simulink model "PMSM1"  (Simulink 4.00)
settings: Solver=ode45  StartTime=-eps  StopTime=0.2  FixedStep=0.000001  RelTol=1e-3
undefined symbols (not defined in the file or in its folder): di, Element, J, Lsx, Lsy, p, Psim, Rs, sfunxy, Symmetrized, Ts, Udc, Warning
libraries: simulink3 x1

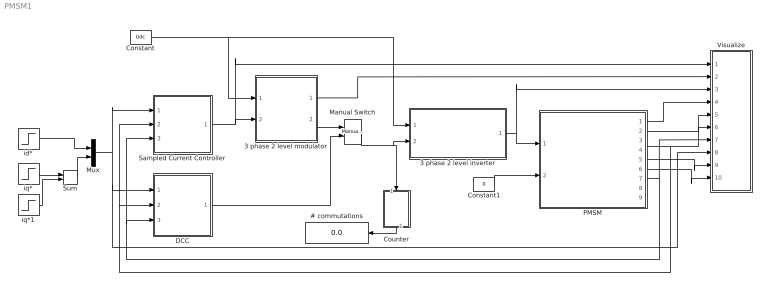
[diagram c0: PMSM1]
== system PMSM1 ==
  # commutations : Display
  3 phase 2 level inverter : Subsystem
  3 phase 2 level modulator : Subsystem  mask{type=Symmetrized, Random=Fixed frequency, Ts=Ts}
      mask prompts: type "Sinus, Symmetrized or Minimum switch modulation"; Random "Fixed or random modulation?"; Ts "Sampling interval"
      mask help: Carrier Wave modulator that uses either fixed frequency modulation or random modulation. The fixed frequency modulation uses 1/(2Ts) as modulation frequency. The random modulation selects the modulatio frequency by random every sampling instant. The selection uses either 1/Ts, 1/(2Ts) or 1/(3Ts) as carrier wave frequency.
  Constant : Constant  Value=Udc
  Constant1 : Constant  Value=0
  Counter : Subsystem  Orientation=down
  DCC : Subsystem
  Manual Switch : simulink3/Nonlinear/Manual Switch  sw=1  action=0
  Mux : Mux  Inputs=2
  PMSM : Subsystem  mask{Psim=Psim, p=p, Rs=Rs, isy=[0 1], psisy=[0 Lsy], isx=[0 1], psisx=[0 Lsx], J=J}
      mask prompts: p "Number of poles"; Rs "Stator resistance"; isy "y-axis current vector"; psisy "y-axis flux vector"; isx "x-axis current vector"; psisx "x-axis flux vector"; J "Inertia"
  Sampled Current Controller : Subsystem  mask{R=Rs, Lx=Lsx, Ly=Lsy, Kp=[(Lsx/Ts+Rs/2) (Lsy/Ts+Rs/2)]', Ti=[(Lsx/Rs+Ts/2) (Lsy/Rs+Ts/2)]', Ts=Ts, Umax=Udc, Umin=-Udc, SlowFast=Fast computer}
      mask prompts: R "Load resistance"; Lx "x-axis load inductance"; Ly "y-axis load inductance"; Kp "Controller gain"; Ti "Integral Time Constant"; Ts "Sampling time [s]"; Umax "Max output signal"; Umin "Min output signal"; SlowFast "Controller type"
  Sum : Sum  Inputs=++  SaturateOnIntegerOverflow=on
  Visualize : Subsystem
  id* : Step  Time=0.0105  Before=0  After=0  SampleTime=0
  iq* : Step  Time=0.0055  Before=0  After=10  SampleTime=0
  iq*1 : Step  Time=0.05  Before=0  After=-5  SampleTime=0
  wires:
  3 phase 2 level inverter/1(va,b,c) -> Visualize/3(v), PMSM/1(vabc)
  Sampled Current Controller/1(u*) -> 3 phase 2 level modulator/2(uabc*), Visualize/1(u*)
  Constant/1 -> 3 phase 2 level inverter/1(Udc), 3 phase 2 level modulator/1(Udc)
  Counter/1(#) -> # commutations/1
  3 phase 2 level modulator/2(sa,b,c) -> Manual Switch/1
  Manual Switch/1 -> 3 phase 2 level inverter/2(sa,b,c), Counter/1(sa,b,c)
  DCC/1(sa,b,c) -> Manual Switch/2
  3 phase 2 level modulator/1(mod) -> Visualize/2(mod)
  id*/1 -> Mux/1
  Mux/1 -> Sampled Current Controller/1(Ref_dq), DCC/1(Ref_dq), Visualize/8(i*dq)
  PMSM/7(theta_el) -> Visualize/7(theta), Sampled Current Controller/3(thetaR), DCC/3(thetaR)
  Constant1/1 -> PMSM/2(Tl)
  PMSM/1(uabc) -> Visualize/4("u ")
  PMSM/4(is) -> Visualize/6(i), DCC/2(Act_ab), Sampled Current Controller/2(Act_ab)
  PMSM/2(exy) -> Visualize/5(e)
  PMSM/5(T_mech) -> Visualize/9(Tmech)
  PMSM/6(w_mech) -> Visualize/10(wmech)
  iq*/1 -> Sum/1
  iq*1/1 -> Sum/2
  Sum/1 -> Mux/2

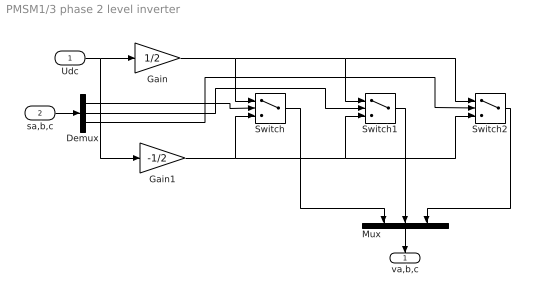
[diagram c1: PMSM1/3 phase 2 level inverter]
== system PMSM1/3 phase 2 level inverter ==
  Udc : Inport  Port=1  LatchInput=off
  sa,b,c : Inport  Port=2  LatchInput=off
  Demux : Demux  Outputs=3  BusSelectionMode=off
  Gain : Gain  Gain=1/2  Multiplication=Element-wise(K.*u)  SaturateOnIntegerOverflow=on
  Gain1 : Gain  Gain=-1/2  Multiplication=Element-wise(K.*u)  SaturateOnIntegerOverflow=on
  Mux : Mux  Orientation=down  Inputs=3
  Switch : Switch  Threshold=0
  Switch1 : Switch  Threshold=0
  Switch2 : Switch  Threshold=0
  va,b,c : Outport  Orientation=down  Port=1  InitialOutput=0
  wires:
  Gain/1 -> Switch/1, Switch1/1, Switch2/1
  Gain1/1 -> Switch/3, Switch1/3, Switch2/3
  Udc/1 -> Gain1/1, Gain/1
  sa,b,c/1 -> Demux/1
  Demux/1 -> Switch/2
  Demux/2 -> Switch1/2
  Demux/3 -> Switch2/2
  Switch/1 -> Mux/1
  Switch1/1 -> Mux/2
  Switch2/1 -> Mux/3
  Mux/1 -> va,b,c/1

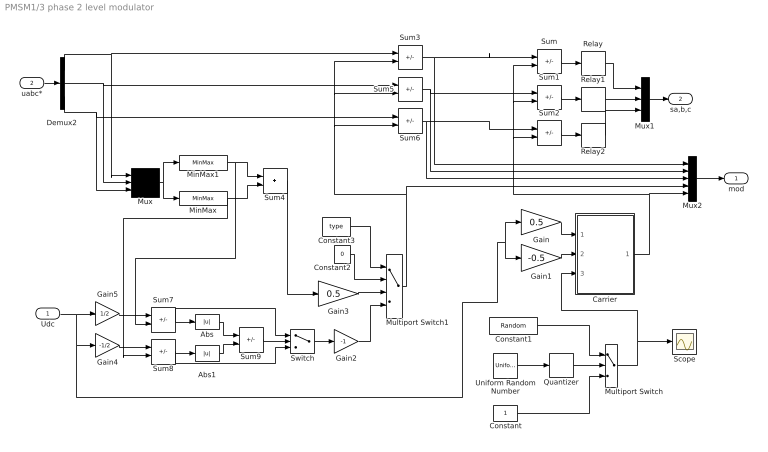
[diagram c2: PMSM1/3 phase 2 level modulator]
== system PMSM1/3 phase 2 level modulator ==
  Udc : Inport  Port=1  LatchInput=off
  uabc* : Inport  Port=2  LatchInput=off
  Abs : Abs  SaturateOnIntegerOverflow=on
  Abs1 : Abs  SaturateOnIntegerOverflow=on
  Carrier : Subsystem
  Constant : Constant  Value=1
  Constant1 : Constant  Value=Random
  Constant2 : Constant  Value=0
  Constant3 : Constant  Value=type
  Demux2 : Demux  Outputs=3  BusSelectionMode=off
  Gain : Gain  Gain=0.5  Multiplication=Element-wise(K.*u)  SaturateOnIntegerOverflow=on
  Gain1 : Gain  Gain=-0.5  Multiplication=Element-wise(K.*u)  SaturateOnIntegerOverflow=on
  Gain2 : Gain  Gain=-1  Multiplication=Element-wise(K.*u)  SaturateOnIntegerOverflow=on
  Gain3 : Gain  Gain=0.5  Multiplication=Element-wise(K.*u)  SaturateOnIntegerOverflow=on
  Gain4 : Gain  Gain=-1/2  Multiplication=Element-wise(K.*u)  SaturateOnIntegerOverflow=on
  Gain5 : Gain  Gain=1/2  Multiplication=Element-wise(K.*u)  SaturateOnIntegerOverflow=on
  MinMax : MinMax  Function=min  Inputs=1
  MinMax1 : MinMax  Function=max  Inputs=1
  Multiport Switch : MultiPortSwitch  Inputs=2
  Multiport Switch1 : MultiPortSwitch  Inputs=3
  Mux : Mux  Inputs=3
  Mux1 : Mux  Inputs=3
  Mux2 : Mux  Inputs=5
  Quantizer : Quantizer  QuantizationInterval=1  LinearizeAsGain=on
  Relay : Relay  OnSwitchValue=eps  OffSwitchValue=eps  OnOutputValue=1  OffOutputValue=-1
  Relay1 : Relay  OnSwitchValue=eps  OffSwitchValue=eps  OnOutputValue=1  OffOutputValue=-1
  Relay2 : Relay  OnSwitchValue=eps  OffSwitchValue=eps  OnOutputValue=1  OffOutputValue=-1
  Scope : Scope
  Sum{,1..3,5..8} (8 alike) : Sum  Inputs=+-  SaturateOnIntegerOverflow=on
  Sum4 : Sum  Inputs=++  SaturateOnIntegerOverflow=on
  Sum9 : Sum  Inputs=-+  SaturateOnIntegerOverflow=on
  Switch : Switch  Threshold=0
  Uniform Random Number : UniformRandomNumber  Minimum=1  Maximum=3  Seed=0.9874  SampleTime=Ts
  mod : Outport  Port=1  InitialOutput=0
  sa,b,c : Outport  Port=2  InitialOutput=0
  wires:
  Carrier/1(um) -> Sum2/2, Sum1/2, Sum/2, Mux2/5
  Gain1/1 -> Carrier/2(Umin)
  Gain/1 -> Carrier/1(Umax)
  Sum/1 -> Relay/1
  Relay1/1 -> Mux1/2
  Sum1/1 -> Relay1/1
  Relay2/1 -> Mux1/3
  Sum2/1 -> Relay2/1
  Quantizer/1 -> Multiport Switch/2
  Uniform Random Number/1 -> Quantizer/1
  Constant/1 -> Multiport Switch/3
  Multiport Switch/1 -> Carrier/3(x), Scope/1
  Constant1/1 -> Multiport Switch/1
  Sum3/1 -> Mux2/1, Sum/1
  Sum5/1 -> Mux2/2, Sum1/1
  Sum6/1 -> Mux2/3, Sum2/1
  Demux2/1 -> Sum3/1, Mux/1
  Demux2/2 -> Sum5/1, Mux/2
  Demux2/3 -> Sum6/1, Mux/3
  Mux/1 -> MinMax1/1, MinMax/1
  MinMax1/1 -> Sum4/1, Sum7/2
  MinMax/1 -> Sum4/2, Sum8/2
  Udc/1 -> Gain5/1, Gain4/1, Gain1/1, Gain/1
  Gain4/1 -> Sum8/1
  Sum7/1 -> Abs/1, Switch/1
  Sum8/1 -> Abs1/1, Switch/3
  Abs/1 -> Sum9/1
  Abs1/1 -> Sum9/2
  Sum9/1 -> Switch/2
  Sum4/1 -> Gain3/1
  Switch/1 -> Gain2/1
  Constant3/1 -> Multiport Switch1/1
  Constant2/1 -> Multiport Switch1/2
  Gain3/1 -> Multiport Switch1/3
  Gain2/1 -> Multiport Switch1/4
  Multiport Switch1/1 -> Sum5/2, Sum3/2, Sum6/2, Mux2/4
  Gain5/1 -> Sum7/1
  uabc*/1 -> Demux2/1
  Relay/1 -> Mux1/1
  Mux1/1 -> sa,b,c/1
  Mux2/1 -> mod/1

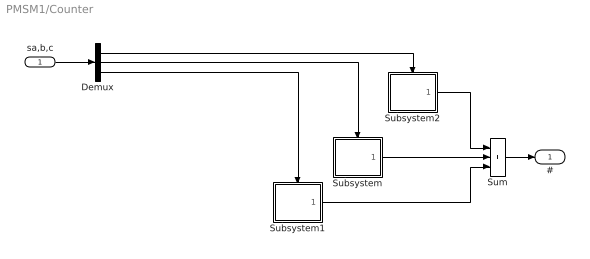
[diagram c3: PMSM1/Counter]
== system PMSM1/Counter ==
  sa,b,c : Inport  Port=1  LatchInput=off
  Demux : Demux  Outputs=3  BusSelectionMode=off
  Subsystem : Subsystem  TreatAsAtomicUnit=on
  Subsystem1 : Subsystem  TreatAsAtomicUnit=on
  Subsystem2 : Subsystem  TreatAsAtomicUnit=on
  Sum : Sum  Inputs=+++  SaturateOnIntegerOverflow=on
  # : Outport  Port=1
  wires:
  Sum/1 -> #/1
  Subsystem/1(Out1) -> Sum/2
  Subsystem2/1(Out1) -> Sum/1
  Subsystem1/1(Out1) -> Sum/3
  sa,b,c/1 -> Demux/1
  Demux/2 -> Subsystem/Trigger
  Demux/3 -> Subsystem1/Trigger
  Demux/1 -> Subsystem2/Trigger

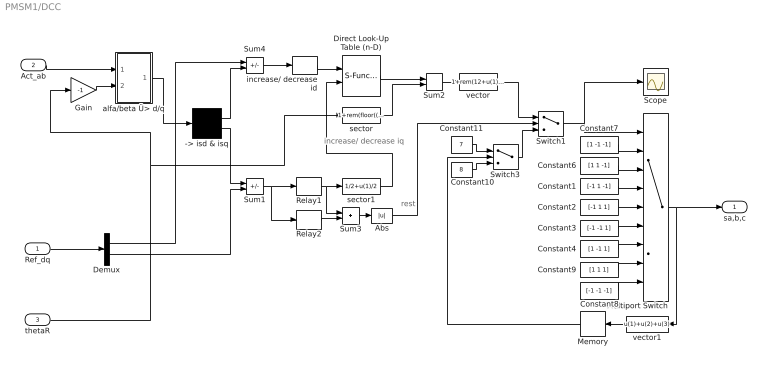
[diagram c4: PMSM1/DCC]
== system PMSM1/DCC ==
  note: increase/ decrease iq
  note: rest
  Ref_dq : Inport  Port=1  LatchInput=off
  Act_ab : Inport  Port=2  LatchInput=off
  thetaR : Inport  Port=3  LatchInput=off
  -> isd & isq : Demux  Outputs=2  BusSelectionMode=off
  Abs : Abs  SaturateOnIntegerOverflow=on
  Constant1 : Constant  Value=[-1 1 -1]
  Constant10 : Constant  Value=8
  Constant11 : Constant  Value=7
  Constant2 : Constant  Value=[-1 1 1]
  Constant3 : Constant  Value=[-1 -1 1]
  Constant4 : Constant  Value=[1 -1 1]
  Constant6 : Constant  Value=[1 1 -1]
  Constant7 : Constant  Value=[1 -1 -1]
  Constant8 : Constant  Value=[-1 -1 -1]
  Constant9 : Constant  Value=[1 1 1]
  Demux : Demux  Outputs=2  BusSelectionMode=off
  Direct Look-Up Table (n-D) : S-Function  FunctionName=sfun_nddirectlook  Parameters=numInputs,mxTable,clipFlag,tabIsInput,numTDims  PortCounts=[]  SFunctionModules=''  mask(LookupNDDirect){maskTabDims=2, explicitNumDims=1, outDims=Element, tabIsInput=off, mxTable=[4 2;5 1], clipFlag=Warning}
      mask prompts: maskTabDims "Number of table dimensions:"; explicitNumDims "Explicit number of table dimensions:"; outDims "Inputs select this object from table:"; tabIsInput "Make table an input"; mxTable "Table data:"; clipFlag "Action for out of range input:"
      mask help: Table member selection. Inputs are zero-based indices into the table, e.g., an input of 3 returns the fourth element in that dimension. Block can also be used to select a column or 2-D matrix out of the table.
      mask init:
      | if tabIsInput == 1
      |   tWhat = ' T';
      |   yT = 1/(3+maskTabDims-outDims);
      | else
      |   tWhat = ' ';
      |   yT = 0;
      | end
      | if maskTabDims >= 5
      |   numTDims = explicitNumDims;
      | else
      |   numTDims = maskTabDims;
      | end
      | numInputs =  numTDims - (outDims-1);
      | if strcmp(get_param(bdroot(gcb),'BlockDiagramType'),'library')
      |   dimsChar = 'n';
      | else
      |   dimsChar = sprintf('%d',numTDims);
      | end
      | [x,y] = nddirectico('plotdata', numTDims, tabIsInput, outDims);
      | xp = x((end-3):end); yp = y((end-3):end);
      | x = x(1:(end-4)); y = y(1:(end-4));
  Gain : Gain  Gain=-1  Multiplication=Element-wise(K.*u)  SaturateOnIntegerOverflow=on
  Memory : Memory  Orientation=left  X0=0  InheritSampleTime=off
  Multiport Switch : MultiPortSwitch  Inputs=8
  Relay1 : Relay  OnSwitchValue=di/2  OffSwitchValue=-di/2  OnOutputValue=1  OffOutputValue=-1
  Relay2 : Relay  OnSwitchValue=1.3*di/2  OffSwitchValue=-1.3*di/2  OnOutputValue=1  OffOutputValue=-1
  Scope : Scope
  Sum1 : Sum  Inputs=-+  SaturateOnIntegerOverflow=on
  Sum2 : Sum  Inputs=++  SaturateOnIntegerOverflow=on
  Sum3 : Sum  Inputs=++  SaturateOnIntegerOverflow=on
  Sum4 : Sum  Inputs=+-  SaturateOnIntegerOverflow=on
  Switch1 : Switch  Threshold=1
  Switch3 : Switch  Threshold=1
  alfa/beta Ü> d/q : Subsystem
  increase/ decrease id : Relay  OnSwitchValue=di/2  OffSwitchValue=-di/2  OnOutputValue=1  OffOutputValue=0
  sector : Fcn  Expr=1+rem(floor((2*pi+u(1)+pi/6)/(pi/3+eps)),6)
  sector1 : Fcn  Expr=1/2+u(1)/2
  vector : Fcn  Expr=1+rem(12+u(1)-1,6)
  vector1 : Fcn  Orientation=left  Expr=u(1)+u(2)+u(3)
  sa,b,c : Outport  Port=1
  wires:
  Gain/1 -> alfa/beta Ü> d/q/2(angle)
  Act_ab/1 -> alfa/beta Ü> d/q/1(vect)
  alfa/beta Ü> d/q/1(Out) -> -> isd & isq/1
  -> isd & isq/1 -> Sum4/2
  Multiport Switch/1 -> vector1/1, sa,b,c/1
  Switch1/1 -> Multiport Switch/1, Scope/1
  vector/1 -> Switch1/1
  Sum4/1 -> increase/ decrease id/1
  Sum2/1 -> vector/1
  vector1/1 -> Memory/1
  -> isd & isq/2 -> Sum1/1
  Constant10/1 -> Switch3/3
  Constant11/1 -> Switch3/1
  Memory/1 -> Switch3/2
  Switch3/1 -> Switch1/3
  Relay1/1 -> Sum3/1, sector1/1
  Relay2/1 -> Sum3/2
  Sum3/1 -> Abs/1
  Sum1/1 -> Relay1/1, Relay2/1
  Abs/1 -> Switch1/2
  increase/ decrease id/1 -> Direct Look-Up Table (n-D)/1
  sector1/1 -> Direct Look-Up Table (n-D)/2
  sector/1 -> Sum2/2
  Direct Look-Up Table (n-D)/1 -> Sum2/1
  Constant6/1 -> Multiport Switch/3
  Constant7/1 -> Multiport Switch/2
  Constant8/1 -> Multiport Switch/9
  Constant9/1 -> Multiport Switch/8
  Constant1/1 -> Multiport Switch/4
  Constant2/1 -> Multiport Switch/5
  Constant3/1 -> Multiport Switch/6
  Constant4/1 -> Multiport Switch/7
  Ref_dq/1 -> Demux/1
  Demux/1 -> Sum4/1
  Demux/2 -> Sum1/2
  thetaR/1 -> Gain/1, sector/1

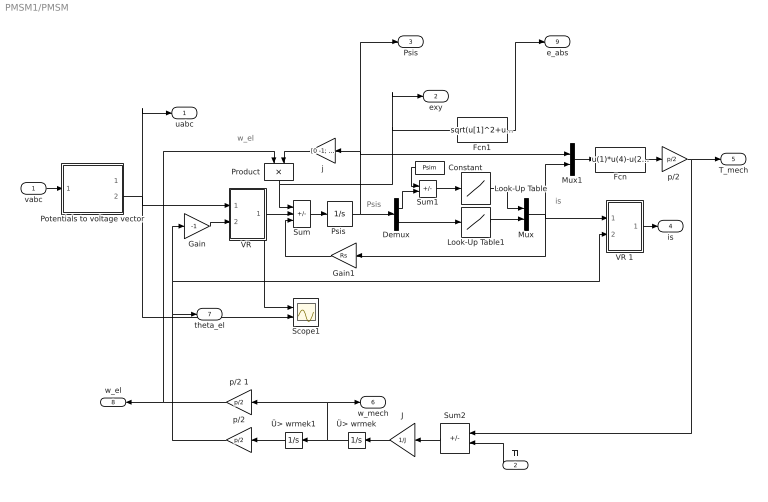
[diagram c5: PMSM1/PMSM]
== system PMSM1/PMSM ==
  note: w_el
  note: Psis
  note: is
  vabc : Inport  Port=1  LatchInput=off
  Tl : Inport  Orientation=left  Port=2  LatchInput=off
  Constant : Constant  Orientation=left  Value=Psim
  Demux : Demux  Outputs=2  BusSelectionMode=off
  Fcn : Fcn  Expr=u(1)*u(4)-u(2)*u(3)
  Fcn1 : Fcn  Expr=sqrt(u[1]^2+u[2]^2)
  Gain : Gain  Gain=-1  Multiplication=Element-wise(K.*u)  SaturateOnIntegerOverflow=on
  Gain1 : Gain  Orientation=left  Gain=Rs  Multiplication=Element-wise(K.*u)  SaturateOnIntegerOverflow=on
  J : Gain  Orientation=left  Gain=1/J  Multiplication=Element-wise(K.*u)  SaturateOnIntegerOverflow=on
  Look-Up Table : Lookup  InputValues=psisx  OutputValues=isx
  Look-Up Table1 : Lookup  InputValues=psisy  OutputValues=isy
  Mux : Mux  Inputs=2
  Mux1 : Mux  Inputs=2
  Potentials to voltage vector : Subsystem
  Product : Product  Orientation=down  Inputs=2  Multiplication=Element-wise(.*)  SaturateOnIntegerOverflow=on
  "Psis " : Integrator  ExternalReset=none  InitialConditionSource=internal  InitialCondition=[Psim 0]'  LimitOutput=on  UpperSaturationLimit=[2*Psim Psim*2]'  LowerSaturationLimit=[Psim/20 0]'  ShowSaturationPort=off  ShowStatePort=off  AbsoluteTolerance=auto
  Scope1 : Scope  NumInputPorts=2
  Sum : Sum  Inputs=-+-  SaturateOnIntegerOverflow=on
  Sum1 : Sum  Inputs=-+  SaturateOnIntegerOverflow=on
  Sum2 : Sum  Orientation=left  Inputs=+-  SaturateOnIntegerOverflow=on
  "VR " : Subsystem
  VR 1 : Subsystem
  j : Gain  Orientation=left  Gain=[0 -1; 1 0]  Multiplication=Matrix(K*u)  SaturateOnIntegerOverflow=on
  p/2 : Gain  Orientation=left  Gain=p/2  Multiplication=Matrix(K*u)  SaturateOnIntegerOverflow=on
  "p/2 " : Gain  Gain=p/2  Multiplication=Matrix(K*u)  SaturateOnIntegerOverflow=on
  p/2 1 : Gain  Orientation=left  Gain=p/2  Multiplication=Matrix(K*u)  SaturateOnIntegerOverflow=on
  Ü> wrmek : Integrator  Orientation=left  ExternalReset=none  InitialConditionSource=internal  InitialCondition=0  LimitOutput=off  UpperSaturationLimit=inf  LowerSaturationLimit=-inf  ShowSaturationPort=off  ShowStatePort=off  AbsoluteTolerance=auto
  Ü> wrmek1 : Integrator  Orientation=left  ExternalReset=none  InitialConditionSource=internal  InitialCondition=0  LimitOutput=off  UpperSaturationLimit=inf  LowerSaturationLimit=-inf  ShowSaturationPort=off  ShowStatePort=off  AbsoluteTolerance=auto
  uabc : Outport  Port=1
  exy : Outport  Port=2
  Psis : Outport  Port=3
  is : Outport  Port=4
  T_mech : Outport  Port=5
  w_mech : Outport  Port=6
  theta_el : Outport  Port=7
  w_el : Outport  Orientation=left  Port=8
  e_abs : Outport  Port=9
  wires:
  VR 1/1(Out) -> is/1
  Ü> wrmek/1 -> Ü> wrmek1/1, p/2 1/1, w_mech/1
  Fcn1/1 -> e_abs/1
  p/2 1/1 -> w_el/1, Product/1
  Tl/1 -> Sum2/2
  Ü> wrmek1/1 -> p/2/1
  Sum2/1 -> J/1
  J/1 -> Ü> wrmek/1
  vabc/1 -> Potentials to voltage vector/1(In1)
  Potentials to voltage vector/2(uab) -> "VR "/1(vect), uabc/1, Scope1/2
  "p/2 "/1 -> Sum2/1, T_mech/1
  Gain/1 -> "VR "/2(angle)
  Sum/1 -> "Psis "/1
  "Psis "/1 -> Demux/1, j/1, Mux1/1, Psis/1
  Demux/1 -> Sum1/2
  Demux/2 -> Look-Up Table1/1
  Look-Up Table/1 -> Mux/1
  Look-Up Table1/1 -> Mux/2
  Mux/1 -> Mux1/2, Gain1/1, VR 1/1(vect)
  Mux1/1 -> Fcn/1
  Constant/1 -> Sum1/1
  Sum1/1 -> Look-Up Table/1
  Gain1/1 -> Sum/3
  "VR "/1(Out) -> Sum/2, Scope1/1
  Product/1 -> Sum/1, Fcn1/1, exy/1
  Fcn/1 -> "p/2 "/1
  j/1 -> Product/2
  p/2/1 -> theta_el/1, Gain/1, VR 1/2(angle)

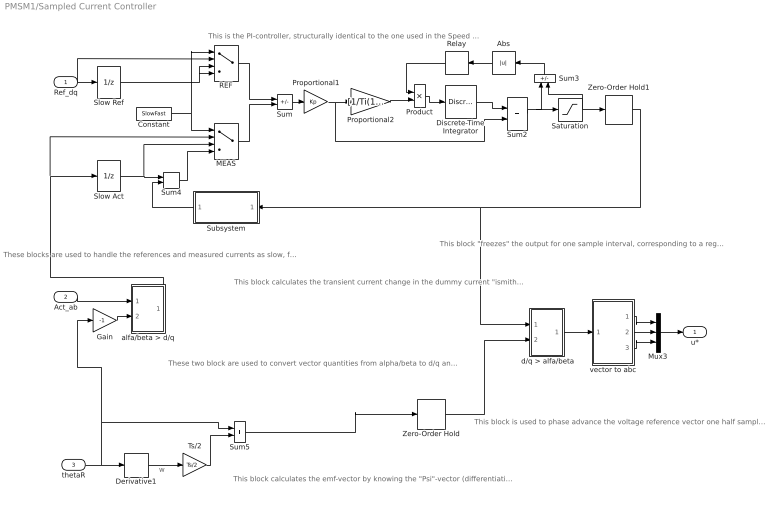
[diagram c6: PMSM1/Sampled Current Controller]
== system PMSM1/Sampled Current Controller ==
  note: These blocks are used to handle the references and measured currents as slow, fast or fast computer with Smith predictor.
  note: This block calculates the transient current change in the dummy current "ismith" The smith predictor calculates the current change that would have been measured if the computer was "fast", i.e. without the delay that a slow computer has. The calculated current change equals the real current change, but informing the controller one sampling interval earlier, thus allowing a high (deadbeat) gain.
  note: This is the PI-controller, structurally identical to the one used in the Speed Controller
  note: This block "freezes" the output for one sample interval, corresponding to a register in a microcontroller where the reference voltages are written once every sampling inteval.
  note: These two block are used to convert vector quantities from alpha/beta to d/q and back again. Note that they are identical, but use the angle with opposite sign.
  note: This block calculates the emf-vector by knowing the "Psi"-vector (differentiation) and calculates the emf- components in the d/q-plane (ideally there is only "eq" whilse "ed"=0). It alse calculates the angle of the "Psi"- vector, used to orient the d/q-plane.
  note: This block is used to phase advance the voltage reference vector one half sample period. It is done to compensate for the fact that the "reality" is turning during the same sample period as the voltage references are being held constant. In the beginning of the sample period, the voltage reference will be 1/2 sample period ahead of reality, and in the end of the sample period it will be 1/2 period behind. In average, it will be in the correct position relative to reality.
  note: w
  Ref_dq : Inport  Port=1  LatchInput=off
  Act_ab : Inport  Port=2  LatchInput=off
  thetaR : Inport  Port=3  LatchInput=off
  " d/q > alfa/beta" : Subsystem
  Abs : Abs  Orientation=left  SaturateOnIntegerOverflow=on
  Constant : Constant  Value=SlowFast
  Derivative1 : Derivative
  Discrete-Time Integrator : DiscreteIntegrator  IntegratorMethod=ForwardEuler  ExternalReset=none  InitialConditionSource=internal  InitialCondition=0  LimitOutput=on  UpperSaturationLimit=Umax  LowerSaturationLimit=Umin  ShowSaturationPort=off  ShowStatePort=off  SampleTime=Ts
  Gain : Gain  Gain=-1  Multiplication=Element-wise(K.*u)  SaturateOnIntegerOverflow=on
  MEAS : MultiPortSwitch  Inputs=3
  Mux3 : Mux  Inputs=3
  Product : Product  Inputs=2  Multiplication=Element-wise(.*)  SaturateOnIntegerOverflow=on
  Proportional1 : Gain  Gain=Kp  Multiplication=Element-wise(K.*u)  SaturateOnIntegerOverflow=on
  Proportional2 : Gain  Gain=[1/Ti(1) 1/Ti(2)]  Multiplication=Element-wise(K.*u)  SaturateOnIntegerOverflow=on
  REF : MultiPortSwitch  Inputs=3
  Relay : Relay  Orientation=left  OnSwitchValue=eps  OffSwitchValue=eps  OnOutputValue=0  OffOutputValue=1
  Saturation : Saturate  UpperLimit=Umax  LowerLimit=Umin  LinearizeAsGain=on
  Slow Act : UnitDelay  X0=0  SampleTime=Ts
  Slow Ref : UnitDelay  X0=0  SampleTime=Ts
  Subsystem : Subsystem  Orientation=left
  Sum : Sum  Inputs=+-  SaturateOnIntegerOverflow=on
  Sum2 : Sum  Inputs=++  SaturateOnIntegerOverflow=on
  Sum3 : Sum  Orientation=up  Inputs=+-  SaturateOnIntegerOverflow=on
  Sum4 : Sum  Inputs=++  SaturateOnIntegerOverflow=on
  Sum5 : Sum  Inputs=++  SaturateOnIntegerOverflow=on
  Ts/2 : Gain  Gain=Ts/2  Multiplication=Matrix(K*u)  SaturateOnIntegerOverflow=on
  Zero-Order Hold : ZeroOrderHold  SampleTime=Ts
  Zero-Order Hold1 : ZeroOrderHold  SampleTime=Ts
  alfa/beta > d/q : Subsystem
  vector to abc : Subsystem
  u* : Outport  Port=1
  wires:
  Discrete-Time Integrator/1 -> Sum2/1
  Proportional1/1 -> Proportional2/1, Sum2/2
  Sum/1 -> Proportional1/1
  Sum2/1 -> Saturation/1, Sum3/1
  Saturation/1 -> Zero-Order Hold1/1, Sum3/2
  Proportional2/1 -> Product/2
  Product/1 -> Discrete-Time Integrator/1
  Relay/1 -> Product/1
  Ref_dq/1 -> REF/2, Slow Ref/1
  Zero-Order Hold1/1 -> Subsystem/1(u), " d/q > alfa/beta"/1(vect)
  Slow Act/1 -> Sum4/1, MEAS/3
  Subsystem/1(di_smith) -> Sum4/2
  Constant/1 -> MEAS/1, REF/1
  Slow Ref/1 -> REF/3, REF/4
  REF/1 -> Sum/1
  Sum4/1 -> MEAS/4
  MEAS/1 -> Sum/2
  Sum3/1 -> Abs/1
  Abs/1 -> Relay/1
  Gain/1 -> alfa/beta > d/q/2(angle)
  Act_ab/1 -> alfa/beta > d/q/1(vect)
  Sum5/1 -> Zero-Order Hold/1
  Zero-Order Hold/1 -> " d/q > alfa/beta"/2(angle)
  " d/q > alfa/beta"/1(Out) -> vector to abc/1(vect)
  vector to abc/1(a) -> Mux3/1
  vector to abc/2(b) -> Mux3/2
  vector to abc/3(c) -> Mux3/3
  alfa/beta > d/q/1(Out) -> Slow Act/1, MEAS/2
  Mux3/1 -> u*/1
  thetaR/1 -> Derivative1/1, Gain/1, Sum5/1
  Derivative1/1 -> Ts/2/1
  Ts/2/1 -> Sum5/2

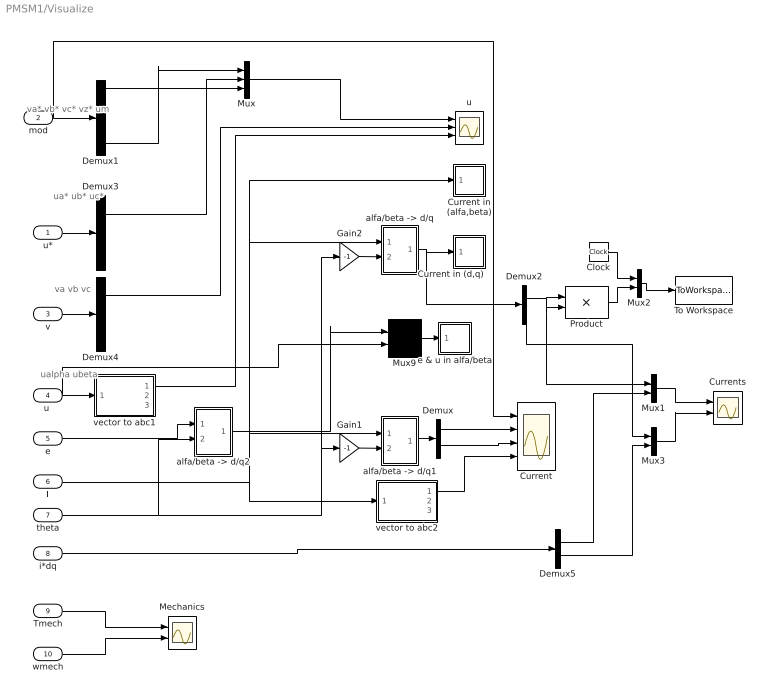
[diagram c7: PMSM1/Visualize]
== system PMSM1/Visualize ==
  note: va* vb* vc* vz* um
  note: ua* ub* uc*
  note: ualpha ubeta
  note: va vb vc
  u* : Inport  Port=1  LatchInput=off
  mod : Inport  Port=2  LatchInput=off
  v : Inport  Port=3  LatchInput=off
  "u " : Inport  Port=4  LatchInput=off
  e : Inport  Port=5  LatchInput=off
  i : Inport  Port=6  LatchInput=off
  theta : Inport  Port=7  LatchInput=off
  i*dq : Inport  Port=8  LatchInput=off
  Tmech : Inport  Port=9  LatchInput=off
  wmech : Inport  Port=10  LatchInput=off
  Clock : Clock
  Current : Scope  NumInputPorts=4
  Current in (alfa,beta) : Subsystem  LoadFcn=sfunxy([],[],[],'LoadBlock')  StartFcn=sfunxy([],[],[],'Start')  StopFcn=sfunxy([],[],[],'Stop')  mask(XY scope.){xmin=-20, xmax=20, ymin=-20, ymax=20, st=-1}
      mask prompts: xmin "x-min:"; xmax "x-max:"; ymin "y-min:"; ymax "y-max:"; st "Sample time:"
      mask help: XY scope using MATLAB graph window. First input is used as time base. Enter plotting ranges.
  Current in (d,q) : Subsystem  LoadFcn=sfunxy([],[],[],'LoadBlock')  StartFcn=sfunxy([],[],[],'Start')  StopFcn=sfunxy([],[],[],'Stop')  mask(XY scope.){xmin=-20, xmax=20, ymin=-20, ymax=20, st=-1}
      mask prompts: xmin "x-min:"; xmax "x-max:"; ymin "y-min:"; ymax "y-max:"; st "Sample time:"
      mask help: XY scope using MATLAB graph window. First input is used as time base. Enter plotting ranges.
  Currents : Scope  NumInputPorts=2
  Demux : Demux  Outputs=2  BusSelectionMode=off
  Demux1 : Demux  Outputs=5  BusSelectionMode=off
  Demux2 : Demux  Outputs=2  BusSelectionMode=off
  Demux3 : Demux  Outputs=3  BusSelectionMode=off
  Demux4 : Demux  Outputs=3  BusSelectionMode=off
  Demux5 : Demux  Outputs=2  BusSelectionMode=off
  Gain1 : Gain  Gain=-1  Multiplication=Element-wise(K.*u)  SaturateOnIntegerOverflow=on
  Gain2 : Gain  Gain=-1  Multiplication=Element-wise(K.*u)  SaturateOnIntegerOverflow=on
  Mechanics : Scope  NumInputPorts=2
  Mux : Mux  Inputs=3
  Mux{1..3,9} (4 alike) : Mux  Inputs=2
  Product : Product  Inputs=2  Multiplication=Element-wise(.*)  SaturateOnIntegerOverflow=on
  To Workspace : ToWorkspace  VariableName=f1  SampleTime=-1  SaveFormat=Array
  "alfa/beta -> d/q" : Subsystem
  "alfa/beta -> d/q1" : Subsystem
  "alfa/beta -> d/q2" : Subsystem
  e & u in alfa/beta : Subsystem  LoadFcn=sfunxy([],[],[],'LoadBlock')  StartFcn=sfunxy([],[],[],'Start')  StopFcn=sfunxy([],[],[],'Stop')  mask(XY scope.){xmin=-300, xmax=300, ymin=-300, ymax=300, st=-1}
      mask prompts: xmin "x-min:"; xmax "x-max:"; ymin "y-min:"; ymax "y-max:"; st "Sample time:"
      mask help: XY scope using MATLAB graph window. First input is used as time base. Enter plotting ranges.
  u : Scope  NumInputPorts=3
  vector to abc1 : Subsystem
  vector to abc2 : Subsystem
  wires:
  Gain2/1 -> "alfa/beta -> d/q"/2(angle)
  Gain1/1 -> "alfa/beta -> d/q1"/2(angle)
  "alfa/beta -> d/q1"/1(Out) -> Demux/1
  Demux/1 -> Current/2
  Demux/2 -> Current/3
  vector to abc2/1(a) -> Current/4
  mod/1 -> Demux1/1, Current/1
  "alfa/beta -> d/q"/1(Out) -> Current in (d,q)/1(xy), Demux2/1
  Demux1/5 -> Mux/1
  Demux1/1 -> Mux/3
  Mux/1 -> u/1
  u*/1 -> Demux3/1
  "u "/1 -> vector to abc1/1(vect), Mux9/2
  Demux3/1 -> Mux/2
  v/1 -> Demux4/1
  Demux4/1 -> u/2
  vector to abc1/1(a) -> u/3
  i/1 -> Current in (alfa,beta)/1(xy), "alfa/beta -> d/q"/1(vect), "alfa/beta -> d/q1"/1(vect), vector to abc2/1(vect)
  Mux9/1 -> e & u in alfa/beta/1(xy)
  theta/1 -> Gain1/1, Gain2/1, "alfa/beta -> d/q2"/2(angle)
  Clock/1 -> Mux2/1
  Product/1 -> Mux2/2
  Mux2/1 -> To Workspace/1
  Demux2/1 -> Product/1, Product/2, Mux1/1
  i*dq/1 -> Demux5/1
  Demux5/1 -> Mux1/2
  Demux2/2 -> Mux3/1
  Demux5/2 -> Mux3/2
  Mux3/1 -> Currents/2
  Mux1/1 -> Currents/1
  e/1 -> "alfa/beta -> d/q2"/1(vect)
  "alfa/beta -> d/q2"/1(Out) -> Mux9/1
  Tmech/1 -> Mechanics/1
  wmech/1 -> Mechanics/2

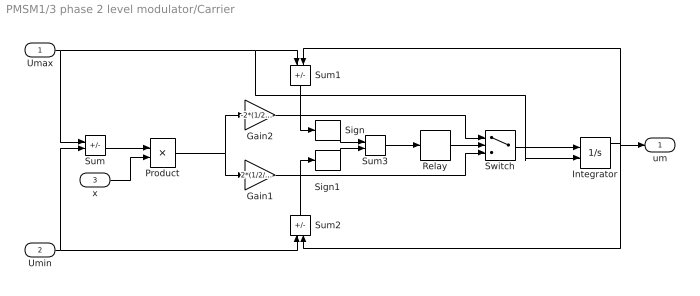
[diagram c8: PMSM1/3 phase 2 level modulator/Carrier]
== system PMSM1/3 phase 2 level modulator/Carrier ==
  Umax : Inport  Port=1  LatchInput=off
  Umin : Inport  Port=2  LatchInput=off
  x : Inport  Port=3  LatchInput=off
  Gain1 : Gain  Gain=2*(1/2/Ts)  Multiplication=Element-wise(K.*u)  SaturateOnIntegerOverflow=on
  Gain2 : Gain  Gain=-2*(1/2/Ts)  Multiplication=Element-wise(K.*u)  SaturateOnIntegerOverflow=on
  Integrator : Integrator  ExternalReset=none  InitialConditionSource=external  InitialCondition=0  LimitOutput=off  UpperSaturationLimit=inf  LowerSaturationLimit=-inf  ShowSaturationPort=off  ShowStatePort=off  AbsoluteTolerance=auto
  Product : Product  Inputs=2  Multiplication=Element-wise(.*)  SaturateOnIntegerOverflow=on
  Relay : Relay  OnSwitchValue=1  OffSwitchValue=-1  OnOutputValue=1  OffOutputValue=-1
  Sign : Signum
  Sign1 : Signum
  Sum : Sum  Inputs=+-  SaturateOnIntegerOverflow=on
  Sum1 : Sum  Orientation=down  Inputs=-+  SaturateOnIntegerOverflow=on
  Sum2 : Sum  Orientation=up  Inputs=-+  SaturateOnIntegerOverflow=on
  Sum3 : Sum  Inputs=++  SaturateOnIntegerOverflow=on
  Switch : Switch  Threshold=0
  um : Outport  Port=1
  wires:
  Switch/1 -> Integrator/1
  Umax/1 -> Sum/1, Sum1/1, Integrator/2
  Umin/1 -> Sum/2, Sum2/1
  Gain2/1 -> Switch/1
  Gain1/1 -> Switch/3
  Integrator/1 -> Sum1/2, um/1, Sum2/2
  Sum1/1 -> Sign/1
  Sum2/1 -> Sign1/1
  Sign/1 -> Sum3/1
  Sign1/1 -> Sum3/2
  Sum3/1 -> Relay/1
  Relay/1 -> Switch/2
  Sum/1 -> Product/1
  Product/1 -> Gain2/1, Gain1/1
  x/1 -> Product/2

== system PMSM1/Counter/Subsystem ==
  Trigger : TriggerPort  TriggerType=either  OutputDataType=auto
  Constant : Constant  Value=1
  Memory : Memory  Orientation=left  X0=0  InheritSampleTime=on
  Sum : Sum  Inputs=++  SaturateOnIntegerOverflow=on
  Out1 : Outport  Port=1
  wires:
  Sum/1 -> Memory/1, Out1/1
  Memory/1 -> Sum/2
  Constant/1 -> Sum/1

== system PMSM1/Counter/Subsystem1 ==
  Trigger : TriggerPort  TriggerType=either  OutputDataType=auto
  Constant : Constant  Value=1
  Memory : Memory  Orientation=left  X0=0  InheritSampleTime=on
  Sum : Sum  Inputs=++  SaturateOnIntegerOverflow=on
  Out1 : Outport  Port=1
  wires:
  Constant/1 -> Sum/1
  Memory/1 -> Sum/2
  Sum/1 -> Memory/1, Out1/1

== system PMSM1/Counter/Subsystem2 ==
  Trigger : TriggerPort  TriggerType=either  OutputDataType=auto
  Constant : Constant  Value=1
  Memory : Memory  Orientation=left  X0=0  InheritSampleTime=on
  Sum : Sum  Inputs=++  SaturateOnIntegerOverflow=on
  Out1 : Outport  Port=1
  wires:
  Sum/1 -> Memory/1, Out1/1
  Memory/1 -> Sum/2
  Constant/1 -> Sum/1

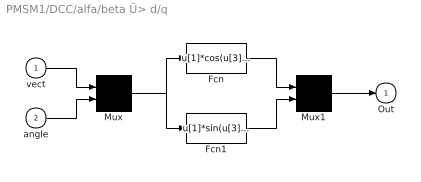
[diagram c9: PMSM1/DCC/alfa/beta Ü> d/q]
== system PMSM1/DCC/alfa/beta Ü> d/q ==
  vect : Inport  Port=1  LatchInput=off
  angle : Inport  Port=2  LatchInput=off
  Fcn : Fcn  Expr=u[1]*cos(u[3])-u[2]*sin(u[3])
  Fcn1 : Fcn  Expr=u[1]*sin(u[3])+u[2]*cos(u[3])
  Mux : Mux  Inputs=2
  Mux1 : Mux  Inputs=2
  Out : Outport  Port=1  InitialOutput=0
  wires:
  vect/1 -> Mux/1
  angle/1 -> Mux/2
  Mux/1 -> Fcn/1, Fcn1/1
  Fcn/1 -> Mux1/1
  Fcn1/1 -> Mux1/2
  Mux1/1 -> Out/1

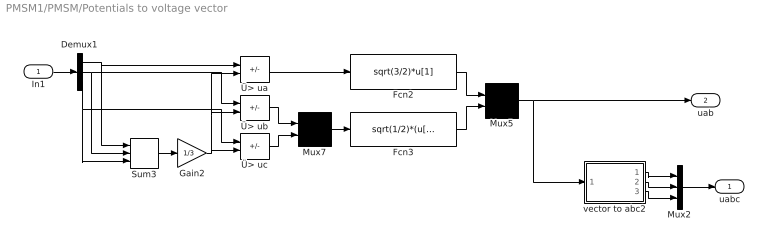
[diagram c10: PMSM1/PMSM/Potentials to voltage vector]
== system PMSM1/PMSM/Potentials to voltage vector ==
  In1 : Inport  Port=1  LatchInput=off
  Demux1 : Demux  Outputs=3  BusSelectionMode=off
  Fcn2 : Fcn  Expr=sqrt(3/2)*u[1]
  Fcn3 : Fcn  Expr=sqrt(1/2)*(u[1]-u[2])
  Gain2 : Gain  Gain=1/3  Multiplication=Element-wise(K.*u)  SaturateOnIntegerOverflow=on
  Mux2 : Mux  Inputs=3
  Mux5 : Mux  Inputs=2
  Mux7 : Mux  Inputs=2
  Sum3 : Sum  Inputs=+++  SaturateOnIntegerOverflow=on
  vector to abc2 : Subsystem
  Ü> ua : Sum  Inputs=+-  SaturateOnIntegerOverflow=on
  Ü> ub : Sum  Inputs=+-  SaturateOnIntegerOverflow=on
  Ü> uc : Sum  Inputs=+-  SaturateOnIntegerOverflow=on
  uabc : Outport  Port=1
  uab : Outport  Port=2
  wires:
  Fcn3/1 -> Mux5/2
  Fcn2/1 -> Mux5/1
  Mux7/1 -> Fcn3/1
  Ü> uc/1 -> Mux7/2
  Ü> ub/1 -> Mux7/1
  Ü> ua/1 -> Fcn2/1
  Gain2/1 -> Ü> uc/2, Ü> ub/2, Ü> ua/2
  Demux1/2 -> Ü> ub/1, Sum3/2
  Sum3/1 -> Gain2/1
  Demux1/3 -> Ü> uc/1, Sum3/3
  Demux1/1 -> Ü> ua/1, Sum3/1
  In1/1 -> Demux1/1
  Mux5/1 -> uab/1, vector to abc2/1(vect)
  vector to abc2/1(a) -> Mux2/1
  vector to abc2/2(b) -> Mux2/2
  vector to abc2/3(c) -> Mux2/3
  Mux2/1 -> uabc/1

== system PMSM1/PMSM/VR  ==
  vect : Inport  Port=1  LatchInput=off
  angle : Inport  Port=2  LatchInput=off
  Fcn : Fcn  Expr=u[1]*cos(u[3])-u[2]*sin(u[3])
  Fcn1 : Fcn  Expr=u[1]*sin(u[3])+u[2]*cos(u[3])
  Mux : Mux  Inputs=2
  Mux1 : Mux  Inputs=2
  Out : Outport  Port=1  InitialOutput=0
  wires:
  Mux1/1 -> Out/1
  Fcn1/1 -> Mux1/2
  Fcn/1 -> Mux1/1
  Mux/1 -> Fcn1/1, Fcn/1
  angle/1 -> Mux/2
  vect/1 -> Mux/1

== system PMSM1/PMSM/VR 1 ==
  vect : Inport  Port=1  LatchInput=off
  angle : Inport  Port=2  LatchInput=off
  Fcn : Fcn  Expr=u[1]*cos(u[3])-u[2]*sin(u[3])
  Fcn1 : Fcn  Expr=u[1]*sin(u[3])+u[2]*cos(u[3])
  Mux : Mux  Inputs=2
  Mux1 : Mux  Inputs=2
  Out : Outport  Port=1  InitialOutput=0
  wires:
  vect/1 -> Mux/1
  angle/1 -> Mux/2
  Mux/1 -> Fcn/1, Fcn1/1
  Fcn/1 -> Mux1/1
  Fcn1/1 -> Mux1/2
  Mux1/1 -> Out/1

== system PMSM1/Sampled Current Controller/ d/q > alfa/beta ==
  vect : Inport  Port=1  LatchInput=off
  angle : Inport  Port=2  LatchInput=off
  Fcn : Fcn  Expr=u[1]*cos(u[3])-u[2]*sin(u[3])
  Fcn1 : Fcn  Expr=u[1]*sin(u[3])+u[2]*cos(u[3])
  Mux : Mux  Inputs=2
  Mux1 : Mux  Inputs=2
  Out : Outport  Port=1  InitialOutput=0
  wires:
  Mux1/1 -> Out/1
  Fcn1/1 -> Mux1/2
  Fcn/1 -> Mux1/1
  Mux/1 -> Fcn1/1, Fcn/1
  angle/1 -> Mux/2
  vect/1 -> Mux/1

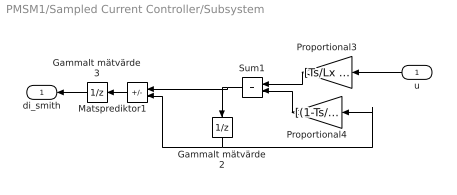
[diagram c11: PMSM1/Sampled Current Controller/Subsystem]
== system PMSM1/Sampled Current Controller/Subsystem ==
  u : Inport  Orientation=left  Port=1  LatchInput=off
  Gammalt mätvärde2 : UnitDelay  Orientation=down  X0=0  SampleTime=Ts
  Gammalt mätvärde3 : UnitDelay  Orientation=left  X0=0  SampleTime=Ts
  Matsprediktor1 : Sum  Orientation=left  Inputs=+-  SaturateOnIntegerOverflow=on
  Proportional3 : Gain  Orientation=left  Gain=[Ts/Lx Ts/Ly]  Multiplication=Element-wise(K.*u)  SaturateOnIntegerOverflow=on
  Proportional4 : Gain  Orientation=left  Gain=[(1-Ts/(Lx/R)) (1-Ts/(Ly/R))]  Multiplication=Element-wise(K.*u)  SaturateOnIntegerOverflow=on
  Sum1 : Sum  Orientation=left  Inputs=++  SaturateOnIntegerOverflow=on
  di_smith : Outport  Orientation=left  Port=1
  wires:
  Proportional3/1 -> Sum1/1
  Proportional4/1 -> Sum1/2
  Sum1/1 -> Gammalt mätvärde2/1, Matsprediktor1/1
  u/1 -> Proportional3/1
  Matsprediktor1/1 -> Gammalt mätvärde3/1
  Gammalt mätvärde3/1 -> di_smith/1
  Gammalt mätvärde2/1 -> Proportional4/1, Matsprediktor1/2

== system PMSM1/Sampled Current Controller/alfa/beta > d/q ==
  vect : Inport  Port=1  LatchInput=off
  angle : Inport  Port=2  LatchInput=off
  Fcn : Fcn  Expr=u[1]*cos(u[3])-u[2]*sin(u[3])
  Fcn1 : Fcn  Expr=u[1]*sin(u[3])+u[2]*cos(u[3])
  Mux : Mux  Inputs=2
  Mux1 : Mux  Inputs=2
  Out : Outport  Port=1  InitialOutput=0
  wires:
  vect/1 -> Mux/1
  angle/1 -> Mux/2
  Mux/1 -> Fcn/1, Fcn1/1
  Fcn/1 -> Mux1/1
  Fcn1/1 -> Mux1/2
  Mux1/1 -> Out/1

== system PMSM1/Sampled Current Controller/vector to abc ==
  vect : Inport  Port=1  LatchInput=off
  Ü> a : Fcn  Expr=sqrt(2/3)*u[1]
  Ü> b : Fcn  Expr=-sqrt(1/6)*u[1]+sqrt(1/2)*u[2]
  Ü> c : Fcn  Expr=-sqrt(1/6)*u[1]-sqrt(1/2)*u[2]
  a : Outport  Port=1  InitialOutput=0
  b : Outport  Port=2  InitialOutput=0
  c : Outport  Port=3  InitialOutput=0
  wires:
  vect/1 -> Ü> b/1, Ü> a/1, Ü> c/1
  Ü> b/1 -> b/1
  Ü> c/1 -> c/1
  Ü> a/1 -> a/1

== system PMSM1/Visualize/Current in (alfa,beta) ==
  xy : Inport  Port=1  LatchInput=off
  sfunxy : S-Function  FunctionName=sfunxy  Parameters=[xmin xmax ymin ymax], st  PortCounts=[]  SFunctionModules=''
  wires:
  xy/1 -> sfunxy/1

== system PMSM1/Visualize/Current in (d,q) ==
  xy : Inport  Port=1  LatchInput=off
  sfunxy : S-Function  FunctionName=sfunxy  Parameters=[xmin xmax ymin ymax], st  PortCounts=[]  SFunctionModules=''
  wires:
  xy/1 -> sfunxy/1

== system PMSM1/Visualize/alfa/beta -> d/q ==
  vect : Inport  Port=1  LatchInput=off
  angle : Inport  Port=2  LatchInput=off
  Fcn : Fcn  Expr=u[1]*cos(u[3])-u[2]*sin(u[3])
  Fcn1 : Fcn  Expr=u[1]*sin(u[3])+u[2]*cos(u[3])
  Mux : Mux  Inputs=2
  Mux1 : Mux  Inputs=2
  Out : Outport  Port=1  InitialOutput=0
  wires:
  vect/1 -> Mux/1
  angle/1 -> Mux/2
  Mux/1 -> Fcn/1, Fcn1/1
  Fcn/1 -> Mux1/1
  Fcn1/1 -> Mux1/2
  Mux1/1 -> Out/1

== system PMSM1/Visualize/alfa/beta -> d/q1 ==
  vect : Inport  Port=1  LatchInput=off
  angle : Inport  Port=2  LatchInput=off
  Fcn : Fcn  Expr=u[1]*cos(u[3])-u[2]*sin(u[3])
  Fcn1 : Fcn  Expr=u[1]*sin(u[3])+u[2]*cos(u[3])
  Mux : Mux  Inputs=2
  Mux1 : Mux  Inputs=2
  Out : Outport  Port=1  InitialOutput=0
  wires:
  Mux1/1 -> Out/1
  Fcn1/1 -> Mux1/2
  Fcn/1 -> Mux1/1
  Mux/1 -> Fcn1/1, Fcn/1
  angle/1 -> Mux/2
  vect/1 -> Mux/1

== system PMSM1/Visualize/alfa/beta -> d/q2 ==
  vect : Inport  Port=1  LatchInput=off
  angle : Inport  Port=2  LatchInput=off
  Fcn : Fcn  Expr=u[1]*cos(u[3])-u[2]*sin(u[3])
  Fcn1 : Fcn  Expr=u[1]*sin(u[3])+u[2]*cos(u[3])
  Mux : Mux  Inputs=2
  Mux1 : Mux  Inputs=2
  Out : Outport  Port=1  InitialOutput=0
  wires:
  vect/1 -> Mux/1
  angle/1 -> Mux/2
  Mux/1 -> Fcn/1, Fcn1/1
  Fcn/1 -> Mux1/1
  Fcn1/1 -> Mux1/2
  Mux1/1 -> Out/1

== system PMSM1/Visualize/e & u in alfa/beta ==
  xy : Inport  Port=1  LatchInput=off
  sfunxy : S-Function  FunctionName=sfunxy4  Parameters=[xmin xmax ymin ymax], st  PortCounts=[]  SFunctionModules=''
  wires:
  xy/1 -> sfunxy/1

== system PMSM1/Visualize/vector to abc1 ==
  vect : Inport  Port=1  LatchInput=off
  Ü> a : Fcn  Expr=sqrt(2/3)*u[1]
  Ü> b : Fcn  Expr=-sqrt(1/6)*u[1]+sqrt(1/2)*u[2]
  Ü> c : Fcn  Expr=-sqrt(1/6)*u[1]-sqrt(1/2)*u[2]
  a : Outport  Port=1  InitialOutput=0
  b : Outport  Port=2  InitialOutput=0
  c : Outport  Port=3  InitialOutput=0
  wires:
  Ü> a/1 -> a/1
  Ü> c/1 -> c/1
  Ü> b/1 -> b/1
  vect/1 -> Ü> c/1, Ü> a/1, Ü> b/1

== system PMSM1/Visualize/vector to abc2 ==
  vect : Inport  Port=1  LatchInput=off
  Ü> a : Fcn  Expr=sqrt(2/3)*u[1]
  Ü> b : Fcn  Expr=-sqrt(1/6)*u[1]+sqrt(1/2)*u[2]
  Ü> c : Fcn  Expr=-sqrt(1/6)*u[1]-sqrt(1/2)*u[2]
  a : Outport  Port=1  InitialOutput=0
  b : Outport  Port=2  InitialOutput=0
  c : Outport  Port=3  InitialOutput=0
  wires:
  vect/1 -> Ü> b/1, Ü> a/1, Ü> c/1
  Ü> b/1 -> b/1
  Ü> c/1 -> c/1
  Ü> a/1 -> a/1

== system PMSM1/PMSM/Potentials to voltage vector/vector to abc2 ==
  vect : Inport  Port=1  LatchInput=off
  Ü> a : Fcn  Expr=sqrt(2/3)*u[1]
  Ü> b : Fcn  Expr=-sqrt(1/6)*u[1]+sqrt(1/2)*u[2]
  Ü> c : Fcn  Expr=-sqrt(1/6)*u[1]-sqrt(1/2)*u[2]
  a : Outport  Port=1  InitialOutput=0
  b : Outport  Port=2  InitialOutput=0
  c : Outport  Port=3  InitialOutput=0
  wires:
  vect/1 -> Ü> b/1, Ü> a/1, Ü> c/1
  Ü> b/1 -> b/1
  Ü> c/1 -> c/1
  Ü> a/1 -> a/1
